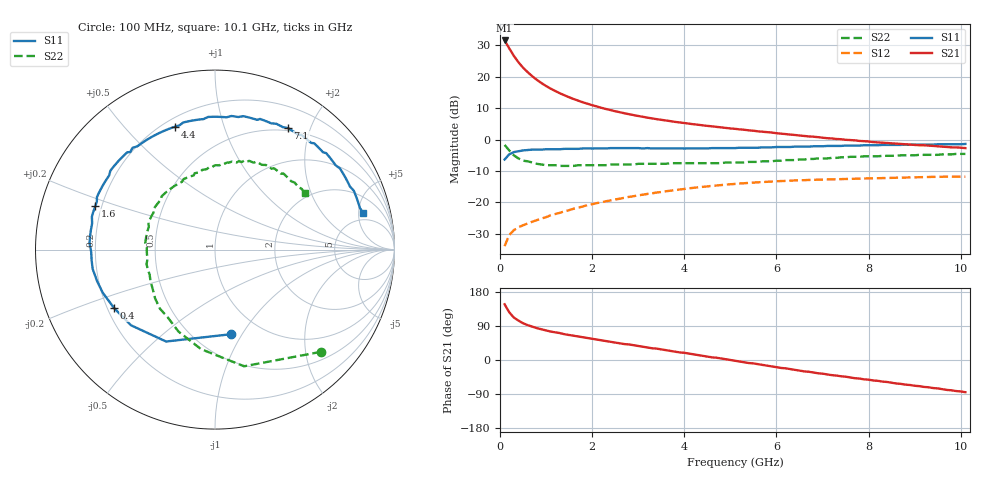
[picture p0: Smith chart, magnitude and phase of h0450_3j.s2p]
!HBFP-0450
!S and NOISE PARAMETERS at Vce=3V  Ic=100mA.  LAST UPDATED  09-04-98
# GHZ S MA R  50
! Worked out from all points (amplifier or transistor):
!   101 points, 100 MHz to 10.1 GHz, reference 50 ohm
!   highest |S21| = 31.6 dB at 100 MHz (marker M1)
!   |S21| within 3 dB of that: start of sweep to 220.6 MHz
!   unconditionally stable (mu >= 1): 2.074 GHz to end of sweep
!   at 1.7 GHz: K = 0.97, MSG = 17.0 dB, |S12| = -21.7 dB
!   at 5.1 GHz: K = 1.09, MAG = 7.0 dB, |S12| = -14.2 dB
!   at 10.1 GHz: K = 1.05, MAG = 3.2 dB, |S12| = -11.8 dB
!   lowest NFmin = 2.34 dB at 1.8 GHz
!   S11 on the Smith chart (normalised r, x): 100 MHz: 0.73, -0.90; 400 MHz: 0.23, -0.26; 1.6 GHz: 0.17, +0.17; 4.4 GHz: 0.25, +0.70; 7.1 GHz: 0.46, +1.67; 10.1 GHz: 3.80, +5.63
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0.1  0.48 -79.0  37.83 147.0  0.02 62.0  0.82 -44.0
0.2  0.58 -118.0  28.34 126.0  0.03 49.0  0.67 -76.0
0.3  0.63 -138.0  21.53 112.0  0.036 43.0  0.56 -98.0
0.4  0.65 -150.0  17.02 104.0  0.04 41.0  0.5 -114.0
0.5  0.67 -159.0  13.96 97.0  0.043 40.0  0.46 -125.0
0.6  0.68 -165.0  11.84 92.0  0.046 40.0  0.45 -133.0
0.7  0.69 -171.0  10.18 88.0  0.049 40.0  0.43 -141.0
0.8  0.69 -175.0  8.92 84.0  0.052 41.0  0.41 -148.0
0.9  0.69 -179.0  7.92 81.0  0.055 42.0  0.4 -154.0
1.1  0.7 174.0  6.46 75.0  0.062 42.0  0.39 -164.0
1.2  0.7 171.0  5.92 73.0  0.065 42.0  0.39 -168.0
1.4  0.71 165.0  5.06 68.0  0.072 42.0  0.38 -176.0
1.6  0.71 160.0  4.41 64.0  0.079 42.0  0.38 178.0
1.8  0.72 156.0  3.91 60.0  0.086 41.0  0.39 172.0
2.5  0.73 141.0  2.82 46.0  0.111 36.0  0.4 157.0
3.5  0.72 124.0  2.06 28.0  0.146 25.0  0.41 139.0
4.4  0.72 108.0  1.68 11.0  0.176 13.0  0.42 123.0
5.1  0.73 95.0  1.48 -2.0  0.196 3.0  0.43 110.0
6.8  0.78 64.0  1.11 -33.0  0.228 -22.0  0.49 81.0
7.1  0.79 59.0  1.05 -38.0  0.231 -26.0  0.5 76.0
8.5  0.82 38.0  0.87 -60.0  0.245 -45.0  0.55 56.0
10.1  0.85 14.0  0.73 -85.0  0.256 -68.0  0.59 32.0
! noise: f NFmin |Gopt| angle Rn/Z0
1.8  2.34  0.69  -147  0.17
2  2.4  0.68  -144  0.2
2.5  2.56  0.69  -135  0.31
3.5  2.87  0.71  -118  0.61
4  3.06  0.72  -108  0.88
5  3.35  0.74  -90  1.5
5.5  3.51  0.77  -80  2
7  3.98  0.8  -54  3.79
8  4.3  0.82  -38  5.37
10  4.93  0.83  -11  8.05
